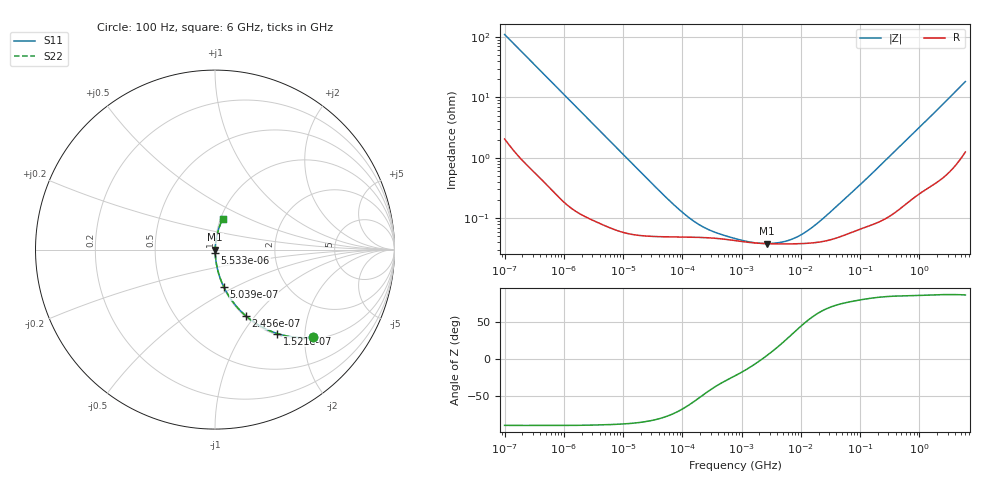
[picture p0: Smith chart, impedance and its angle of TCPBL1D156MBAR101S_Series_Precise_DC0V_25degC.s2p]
! TCPBL1D156MBAR101S Polymer Tantalum Capacitor Sparameter Model
! Model Generated by Samsung Electro-Mechanics
! Samsung Sparameter Version 5.0
! Date : Oct-21-2025
! Products : Polymer Tantalum Capacitor
! Characteristics :
!  Nominal Capacitance = 15uF
!  Capacitance Tolerance = +/-20%
!  ESR = 100 mohm max at 100kHz
!  Rated Voltage = 20Vdc
!  Size = 1411(unit:inch), 3528(unit:mm)
!  Length = 3.50+/-0.20mm
!  Width = 2.80+/-0.20mm
!  Thickness = 0.90+/-0.10mm
!  Lineup = Conductive Polymer Type
!  Feature = PBL
!  Measurement Temperature : 25degC.
!  DC bias Value = 0V
!  Frequency : 100Hz ~ 6GHz
! External Node Assignments :
!  1  o---||---o  2
# MHz S RI R 50.0
! Freq.  Real(S11)  Im(S11)  Real(S12)  Im(S12)  Real(S21)  Im(S21)  Real(S22)  Im(S22)
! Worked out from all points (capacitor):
!   300 points, 100 Hz to 6 GHz, reference 50 ohm
!   read as one part in series: C = 14.5 uF near 106.2 Hz
!   lowest |Z| = 38.1 mohm at 2.645 MHz (marker M1)
!   series resonance near 2.22 MHz, so ESL is about 360 pH
!   S11 on the Smith chart (normalised r, x): 100 Hz: 1.04, -2.19; 152.1 Hz: 1.02, -1.45; 245.6 Hz: 1.01, -0.90; 503.9 Hz: 1.01, -0.44; 5.533 kHz: 1.00, -0.04; 6 GHz: 1.02, +0.36
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0.0001  0.5454 -0.4887  0.4546 0.4887  0.4546 0.4887  0.5454 -0.4887
0.0001520888  0.3464 -0.4675  0.6536 0.4675  0.6536 0.4675  0.3464 -0.4675
0.0002455886  0.1725 -0.3697  0.8275 0.3697  0.8275 0.3697  0.1725 -0.3697
0.0005039354  0.0497 -0.2092  0.9503 0.2092  0.9503 0.2092  0.0497 -0.2092
0.0009739296  0.0149 -0.113  0.9851 0.113  0.9851 0.113  0.0149 -0.113
0.001998454  0.00428 -0.056  0.9957 0.056  0.9957 0.056  0.00428 -0.056
0.005532612  0.00114 -0.0205  0.9989 0.0205  0.9989 0.0205  0.00114 -0.0205
0.03993819  0.000504 -0.00286  0.9995 0.00286  0.9995 0.00286  0.000504 -0.00286
0.09238102  0.00049 -0.00125  0.9995 0.00125  0.9995 0.00125  0.00049 -0.00125
0.17854  0.000483 -0.00066  0.9995 0.00066  0.9995 0.00066  0.000483 -0.00066
0.3249932  0.000469 -0.000383  0.9995 0.000383  0.9995 0.000383  0.000469 -0.000383
0.7981464  0.000424 -0.000171  0.9996 0.000171  0.9996 0.000171  0.000424 -0.000171
1.542536  0.000392 -5.95e-05  0.9996 5.95e-05  0.9996 5.95e-05  0.000392 -5.95e-05
2.644602  0.00038 2.95e-05  0.9996 -2.95e-05  0.9996 -2.95e-05  0.00038 2.95e-05
4.270427  0.000376 0.00012  0.9996 -0.00012  0.9996 -0.00012  0.000376 0.00012
6.895764  0.000376 0.000239  0.9996 -0.000239  0.9996 -0.000239  0.000376 0.000239
10.48768  0.000381 0.000387  0.9996 -0.000387  0.9996 -0.000387  0.000381 0.000387
15.95059  0.000391 0.000602  0.9996 -0.000602  0.9996 -0.000602  0.000391 0.000602
71.30563  0.000587 0.00257  0.9994 -0.00257  0.9994 -0.00257  0.000587 0.00257
318.7652  0.0012 0.0106  0.9988 -0.0106  0.9988 -0.0106  0.0012 0.0106
1922.593  0.0073 0.0587  0.9927 -0.0587  0.9927 -0.0587  0.0073 0.0587
6000  0.0433 0.1722  0.9567 -0.1722  0.9567 -0.1722  0.0433 0.1722
